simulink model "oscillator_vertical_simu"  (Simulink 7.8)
settings: Solver=ode45  StartTime=0.0  StopTime=10.0  RelTol=1e-3
undefined symbols (not defined in the file or in its folder): MP

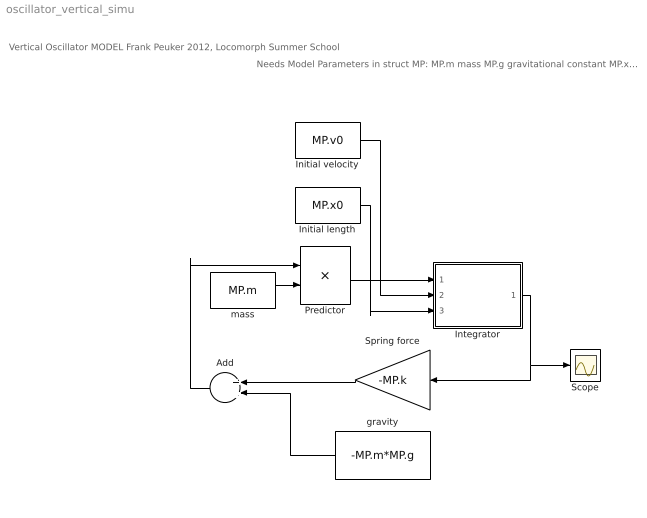
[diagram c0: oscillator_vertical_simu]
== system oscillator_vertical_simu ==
  note: Vertical Oscillator MODEL Frank Peuker 2012, Locomorph Summer School
  note: Needs Model Parameters in struct MP: MP.m mass MP.g gravitational constant MP.x0 initial position MP.v0 initial speed MP.k stiffness of spring
  Add : Sum
  Initial length : Constant  Value=MP.x0
  Initial velocity : Constant  Value=MP.v0
  Integrator : Subsystem
  Predictor : Product  Inputs=*/
  Scope : Scope
  Spring force : Gain  Gain=-MP.k
  gravity : Constant  Value=-MP.m*MP.g
  mass : Constant  Value=MP.m
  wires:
  Initial velocity/1 -> Integrator/2(v_init)
  Initial length/1 -> Integrator/3(L_init)
  Predictor/1 -> Integrator/1(a)
  mass/1 -> Predictor/2
  Integrator/1(L) -> Spring force/1, Scope/1
  Add/1 -> Predictor/1
  gravity/1 -> Add/2
  Spring force/1 -> Add/1

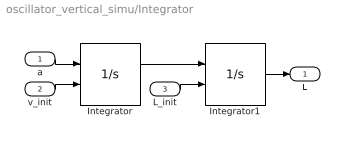
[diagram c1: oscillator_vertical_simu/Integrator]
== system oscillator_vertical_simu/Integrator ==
  a : Inport
  v_init : Inport  Port=2
  L_init : Inport  Port=3
  Integrator : Integrator  InitialConditionSource=external
  Integrator1 : Integrator  InitialConditionSource=external
  L : Outport
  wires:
  Integrator/1 -> Integrator1/1
  a/1 -> Integrator/1
  Integrator1/1 -> L/1
  v_init/1 -> Integrator/2
  L_init/1 -> Integrator1/2
